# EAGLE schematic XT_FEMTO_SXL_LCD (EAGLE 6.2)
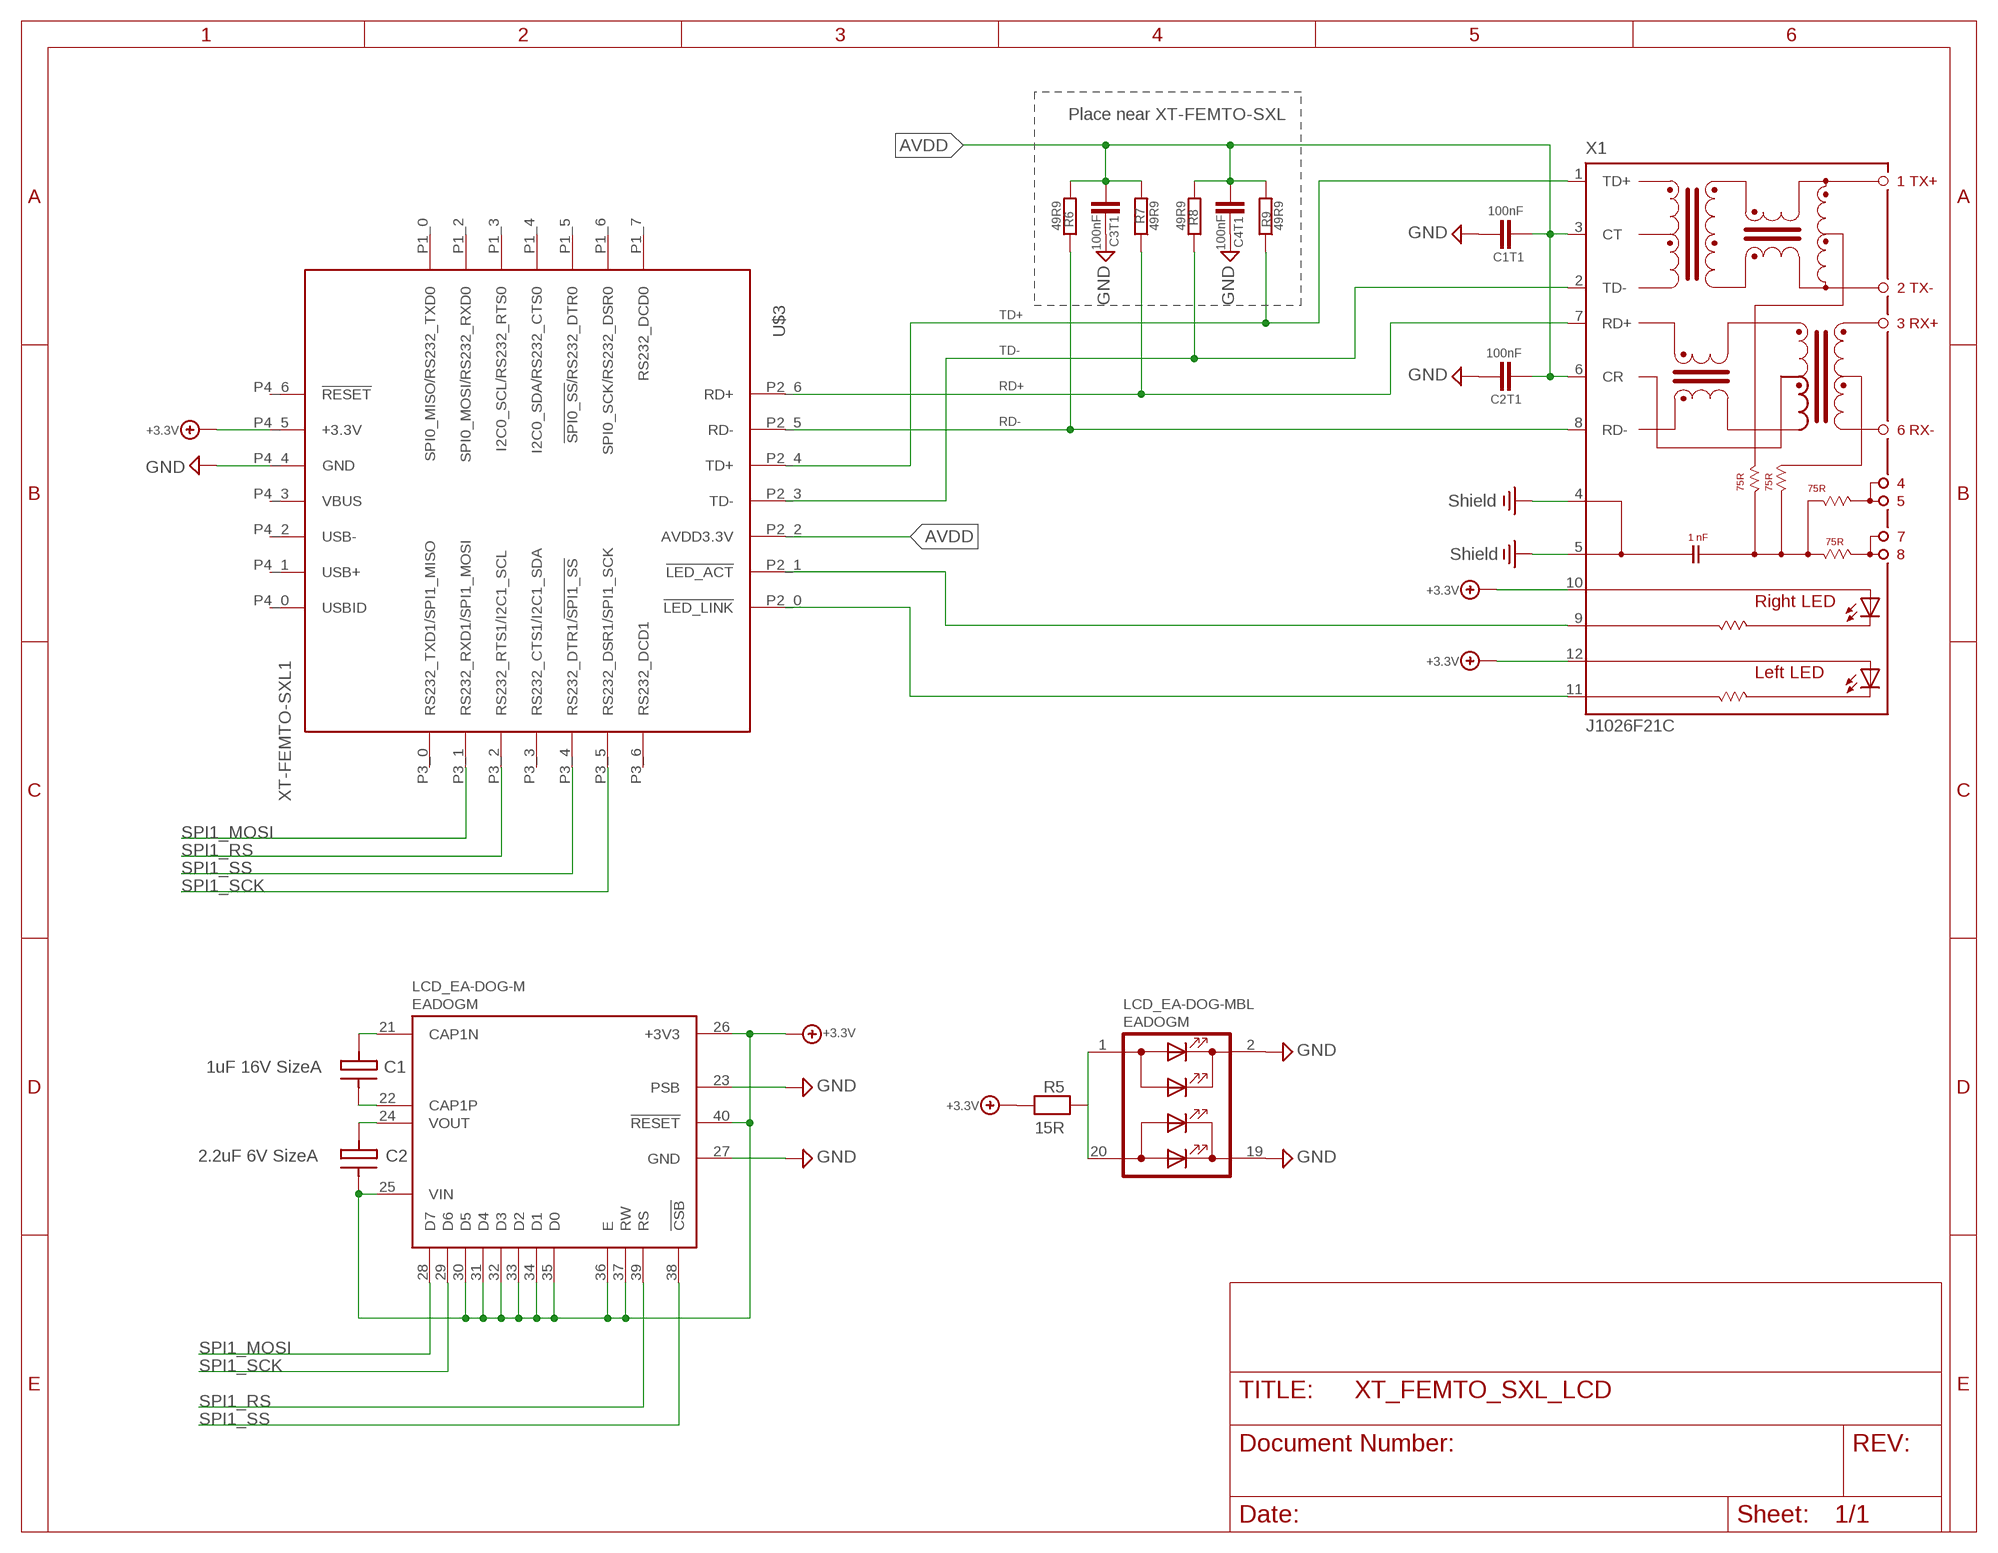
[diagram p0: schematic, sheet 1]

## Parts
C1  1uF 16V SizeA  C3216  [ORCAD_X_CT3216]
C1T1  100nF  CHIP-C-VTS0402  [R0402_VTS]
C2  2.2uF 6V SizeA  C3216  [ORCAD_X_CT3216]
C2T1  100nF  CHIP-C-VTS0402  [R0402_VTS]
C3T1  100nF  CHIP-C-VTS0402  [R0402_VTS]
C4T1  100nF  CHIP-C-VTS0402  [R0402_VTS]
LCD_EA-DOG-M  EADOGM  [EADOGM]
R5  15R  CHIP-R-0603  [SMD-0603@1]
R6  49R9  R-EU_R0603  [R0603]
R7  49R9  R-EU_R0603  [R0603]
R8  49R9  R-EU_R0603  [R0603]
R9  49R9  R-EU_R0603  [R0603]
U$3  XT-FEMTO-SXL1  [XT-FEMTO-SXL-PIN]
X1  J1026F21C  [J1]

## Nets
+3.3V: C2.2(C-) LCD_EA-DOG-M.25(VIN) LCD_EA-DOG-M.26(+3V3) LCD_EA-DOG-M.30(D5) LCD_EA-DOG-M.31(D4) LCD_EA-DOG-M.32(D3) LCD_EA-DOG-M.33(D2) LCD_EA-DOG-M.34(D1) LCD_EA-DOG-M.35(D0) LCD_EA-DOG-M.36(E) LCD_EA-DOG-M.37(RW) LCD_EA-DOG-M.40(!RESET) R5.1 U$3.P4_5(+3.3V) X1.10(A-R) X1.12(A-L)
AVDD: C1T1.1 C2T1.2 C3T1.1 C4T1.2 R6.2 R7.2 R8.2 R9.2 U$3.P2_2(AVDD3.3V) X1.3(CT) X1.6(CR)
GND: C1T1.2 C2T1.1 C3T1.2 C4T1.1 LCD_EA-DOG-M.2(C1) LCD_EA-DOG-M.19(C2) LCD_EA-DOG-M.23(PSB) LCD_EA-DOG-M.27(GND) U$3.P4_4(GND)
N$3: U$3.P2_1(!LED_ACT) X1.9(C-R)
N$5: LCD_EA-DOG-M.1(A1) LCD_EA-DOG-M.20(A2) R5.2
N$7: C2.1(C+) LCD_EA-DOG-M.24(VOUT)
N$8: U$3.P2_0(!LED_LINK) X1.11(C-L)
N$9: C1.2(C-) LCD_EA-DOG-M.22(CAP1P)
N$11: C1.1(C+) LCD_EA-DOG-M.21(CAP1N)
PE: X1.4 X1.5 ; supply symbol labelled Shield
RD+: R7.1 U$3.P2_6(RD+) X1.7(RD+)
RD-: R6.1 U$3.P2_5(RD-) X1.8(RD-)
SPI1_MOSI: LCD_EA-DOG-M.28(D7) U$3.P3_1(RS232_RXD1/SPI1_MOSI)
SPI1_RS: LCD_EA-DOG-M.39(RS) U$3.P3_2(RS232_RTS1/I2C1_SCL)
SPI1_SCK: LCD_EA-DOG-M.29(D6) U$3.P3_5(RS232_DSR1/SPI1_SCK)
SPI1_SS: LCD_EA-DOG-M.38(!CSB) U$3.P3_4(RS232_DTR1/!SPI1_SS!)
TD+: R9.1 U$3.P2_4(TD+) X1.1(TD+)
TD-: R8.1 U$3.P2_3(TD-) X1.2(TD-)
Unconnected: U$3.P1_0(SPI0_MISO/RS232_TXD0) U$3.P1_2(SPI0_MOSI/RS232_RXD0) U$3.P1_3(I2C0_SCL/RS232_RTS0) U$3.P1_4(I2C0_SDA/RS232_CTS0) U$3.P1_5(!SPI0_SS!/RS232_DTR0) U$3.P1_6(SPI0_SCK/RS232_DSR0) U$3.P1_7(RS232_DCD0) U$3.P3_0(RS232_TXD1/SPI1_MISO) U$3.P3_3(RS232_CTS1/I2C1_SDA) U$3.P3_6(RS232_DCD1) U$3.P4_0(USBID) U$3.P4_1(USB+) U$3.P4_2(USB-) U$3.P4_3(VBUS) U$3.P4_6(!RESET)

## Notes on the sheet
- Place near XT-FEMTO-SXL

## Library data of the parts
C1 C2 = XTMACRO:C3216
C1T1 C2T1 C3T1 C4T1 = mea-lib:CHIP-C-?: Chip capacitance
LCD_EA-DOG-M = XTMACRO:EADOGM: THT EA LCD Display With LED Backlight
R5 = mea-lib:CHIP-R-?: Chip resistors
R6-R9 = rcl:R-EU_: RESISTOR, European symbol
U$3 = ak-devices:XT-FEMTO-SXL: AK-NORD XT-FEMTO-SXL
X1 = con-pulse:J1026F: PULSEJACK (TM) 1x1 Tab-UP RJ45 10/100 Base-TX RJ45 1x1 Tab-UP with LEDs 8-pin (J1 series) and 6-pin (JP series) integrated magnetics connector, designed to support applications, such as ADSL modems, LAN-on-Motherboard, and Hub and Switches. Source: www.pulseeng.com .. PulseJack-J402.pdf; OC_FARNELL: unknown; OC_NEWARK: unknown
